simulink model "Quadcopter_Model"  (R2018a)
settings: Solver=VariableStepAuto  StartTime=0.0  StopTime=runtime  FixedStep=0.001  RelTol=1e-3
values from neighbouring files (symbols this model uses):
  delta_T = [ 0,  0,  9.404e-04 ]    [modelParameters.m]    (also in rich_params.m = [ 0,  0,  1.176e-04 ])
  g = 9.81    [modelParameters.m]    (also in rich_params.m)
  height_controlled_o = (((Rm*If        + (((omega0_o * 2 * Rm * Kv * Kq      * Kd + 1)^2) - 1)/(4* Rm*Kv^2*Kq      * Kd))/Vb)*(Pmax - Pmin) + Pmin)    [modelParameters.m]    (also in rich_params.m)
  If = 0.3836    [modelParameters.m]    (also in rich_params.m = 0.39)
  Jreq = 4.2012e-05    [modelParameters.m]    (also in rich_params.m = 1.376e-05)
  Jxx = 0.0110    (= 0.011)    [modelParameters.m]    (also in rich_params.m = 0.0081)
  Jyy = 0.0116    [modelParameters.m]    (also in rich_params.m = 0.0074)
  Jzz = 0.0223    [modelParameters.m]    (also in rich_params.m = 0.0135)
  Kd = 1.4852e-07    [modelParameters.m]    (also in rich_params.m = 5.194e-07)
  Kh = 3.4574e-04    (= 0.00034574)    [modelParameters.m]    (also in rich_params.m)
  Kq = 96.3422    [modelParameters.m]    (also in rich_params.m = 110)
  Kt = 1.2007e-05    [modelParameters.m]    (also in rich_params.m = 7.3956e-06)
  Kv = 96.3422    [modelParameters.m]    (also in rich_params.m = 110)
  m = 1.216    [modelParameters.m]    (also in rich_params.m = 0.656)
  omega0_o = sqrt((m*g)/(4*Kt))    [modelParameters.m]    (also in rich_params.m)
  omega1_o = sqrt((m*g)/(4*Kt))    [modelParameters.m]    (also in rich_params.m)
  omega2_o = sqrt((m*g)/(4*Kt))    [modelParameters.m]    (also in rich_params.m)
  omega3_o = sqrt((m*g)/(4*Kt))    [modelParameters.m]    (also in rich_params.m)
  pitch_o = 0    [modelParameters.m]    (also in rich_params.m)
  pitchrate_o = 0    [modelParameters.m]    (also in rich_params.m)
  Pmax = 1    [modelParameters.m]    (also in rich_params.m)
  Pmin = 0    [modelParameters.m]    (also in rich_params.m)
  r_oc = [ 0 ; 0 ; 0 ]    [modelParameters.m]    (also in rich_params.m)
  rhx = 0.16    [modelParameters.m]    (also in rich_params.m = 0.115)
  rhy = 0.16    [modelParameters.m]    (also in rich_params.m = 0.115)
  rhz = 0.03    [modelParameters.m]    (also in rich_params.m = 0.04)
  Rm = 0.235    [modelParameters.m]    (also in rich_params.m = 0.19)
  roll_o = 0    [modelParameters.m]    (also in rich_params.m)
  rollrate_o = 0    [modelParameters.m]    (also in rich_params.m)
  signal_mixer = [ 1, -1, -1, -1    [modelParameters.m]    (also in rich_params.m)
  Tc = 0.01    [modelParameters.m]    (also in rich_params.m)
  Tq = 0.005    [modelParameters.m]    (also in rich_params.m)
  Vb = 12.3    [modelParameters.m]    (also in rich_params.m = 11.4)
  x_controlled_o = 0    [modelParameters.m]    (also in rich_params.m)
  x_o = 0    [modelParameters.m]    (also in rich_params.m)
  x_vel_o = 0    [modelParameters.m]    (also in rich_params.m)
  y_controlled_o = 0    [modelParameters.m]    (also in rich_params.m)
  y_o = 0    [modelParameters.m]    (also in rich_params.m)
  y_vel_o = 0    [modelParameters.m]    (also in rich_params.m)
  yaw_controlled_o = 0    [modelParameters.m]    (also in rich_params.m)
  yaw_o = 0    [modelParameters.m]    (also in rich_params.m)
  yawrate_o = 0    [modelParameters.m]    (also in rich_params.m)
  z_o = 0    [modelParameters.m]    (also in rich_params.m)
  z_vel_o = 0    [modelParameters.m]    (also in rich_params.m)
undefined symbols (not defined in the file or in its folder): lqr_K
libraries: simulink x16, Derivative x13, dsparch4 x3, vrlib x1
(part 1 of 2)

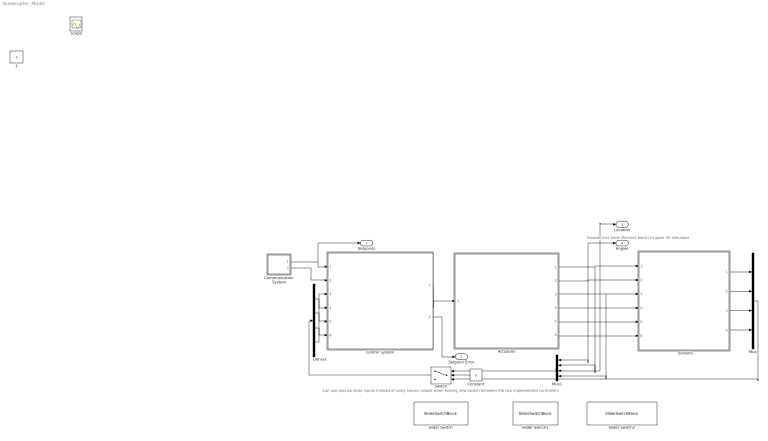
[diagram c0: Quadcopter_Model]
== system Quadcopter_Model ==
  note: Double-click here (Sensors block) to open 3D simulator
  note: Can use precise state inputs instead of noisy sensor values when testing new controls
  note: Switch between the two implemented controllers
  "     Sensors   " : Subsystem
  Actuation : Subsystem
  Communication System : Subsystem
  Constant : Constant  Value=0
  Control System : Subsystem
  Demux : Demux
  Mux : Mux
  Mux1 : Mux
  Slider Switch : SliderSwitchBlock  WebBlockId=752  LabelPosition=Hide
  Slider Switch1 : SliderSwitchBlock  WebBlockId=751  LabelPosition=Hide
  Slider Switch2 : SliderSwitchBlock  WebBlockId=769  LabelPosition=Hide
  Switch : Switch  Criteria=u2 ~= 0
  Setpoint Error : Outport  SignalName=setpoint_error
  Setpoints : Outport  Port=2
  Location : Outport  Port=3
  Angles : Outport  Port=4
  1 : Constant  IOType=siggen
  Scope : Scope
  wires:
  Control System/1(P) -> Actuation/1(P)
  Actuation/6(B_g) -> 1/6
  Actuation/5(B_vo_dot) -> 1/5
  Actuation/1(B_omega) -> Mux1/2, 1/1
  Actuation/2(euler_angles) -> Angles/1, 1/2, Mux1/1
  Communication System/1(Autonomous Setpoints) -> Control System/1(setpoints), Setpoints/1
  Actuation/3(B_vo) -> 1/3, Mux1/4
  1/2 -> Mux/2
  1/1 -> Mux/1
  1/3 -> Mux/3
  Mux/1 -> Switch/3
  Mux1/1 -> Switch/1
  Demux/4 -> Control System/3(velocity)
  Demux/3 -> Control System/6(current_position)
  Demux/2 -> Control System/5(euler_rates)
  Demux/1 -> Control System/4(euler_angles_filtered)
  Switch/1 -> Demux/1
  Constant/1 -> Switch/2
  1/4 -> Mux/4
  Actuation/4(E_ro) -> Location/1, 1/4, Mux1/3
  Control System/2(setpoint error) -> Setpoint Error/1
  Communication System/2(RC commands) -> Control System/2(RC Commands)

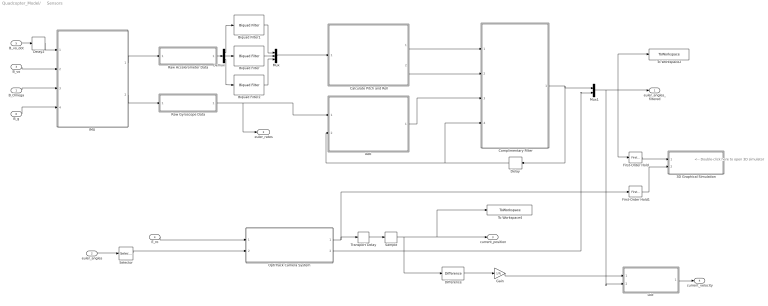
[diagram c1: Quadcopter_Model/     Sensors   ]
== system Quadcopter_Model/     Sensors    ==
  note: <-- Double-click here to open 3D simulator
  B_Omega : Inport
  euler_angles : Inport  Port=2
  B_vo : Inport  Port=3
  E_ro : Inport  Port=4
  B_vo_dot : Inport  Port=5
  B_g : Inport  Port=6
  3D Graphical Simulation : Subsystem
  "Aeb " : MATLAB Function  TreatAsAtomicUnit=on
  Biquad Filter : dsparch4/Biquad Filter  IIRFiltStruct=Direct form II  CoeffSource=Specify via dialog  BiQuadCoeffs=accel_SOS_Matrix  a0Flag=Warning  IC=0  ICnum=0  ICden=0  InputProcessing=Columns as channels (frame based)  denAccumFracLength=30  denProdOutputFracLength=30  secondMemoryFracLength=15  roundingMode=Floor  overflowMode=off  ScaleValues=1  optimizeScaleValues=on  ScaleValueMode=Specify via input port (g)  scaleValueFracLength=14  FilterSource=Specify via dialog  FilterObject=BQF
  Biquad Filter1 : dsparch4/Biquad Filter  IIRFiltStruct=Direct form II  CoeffSource=Specify via dialog  BiQuadCoeffs=accel_SOS_Matrix  a0Flag=Warning  IC=0  ICnum=0  ICden=0  InputProcessing=Columns as channels (frame based)  denAccumFracLength=30  denProdOutputFracLength=30  secondMemoryFracLength=15  roundingMode=Floor  overflowMode=off  ScaleValues=1  optimizeScaleValues=on  ScaleValueMode=Specify via input port (g)  scaleValueFracLength=14  FilterSource=Specify via dialog  FilterObject=BQF
  Biquad Filter2 : dsparch4/Biquad Filter  IIRFiltStruct=Direct form II  CoeffSource=Specify via dialog  BiQuadCoeffs=accel_SOS_Matrix  a0Flag=Warning  IC=0  ICnum=0  ICden=0  InputProcessing=Columns as channels (frame based)  denAccumFracLength=30  denProdOutputFracLength=30  secondMemoryFracLength=15  roundingMode=Floor  overflowMode=off  ScaleValues=1  optimizeScaleValues=on  ScaleValueMode=Specify via input port (g)  scaleValueFracLength=14  FilterSource=Specify via dialog  FilterObject=BQF
  Calculate Pitch and Roll : MATLAB Function  TreatAsAtomicUnit=on
  Complimentary Filter : MATLAB Function  TreatAsAtomicUnit=on
  Delay : Delay  DelayLength=1  InitialCondition=0
  Delay2 : Delay  DelayLength=1  InitialCondition=0  SampleTime=Tq
  Demux : Demux  Outputs=3
  Difference : simulink/Discrete/Difference  ICPrevInput=0.0  OutMin=[]  OutMax=[]  OutDataType=fixdt(1, 16)  OutScaling=2^-10  DoSatur=off
  First-Order Hold : simulink/Discrete/First-Order Hold  DisableCoverage=on  Ts=5e-3
  First-Order Hold1 : simulink/Discrete/First-Order Hold  DisableCoverage=on  Ts=5e-3
  Gain : Gain  Gain=1/Tc
  "IMU " : Subsystem
  "Lbe " : MATLAB Function  TreatAsAtomicUnit=on
  Mux : Mux  Inputs=3
  Mux1 : Mux  Inputs=2
  "OptiTrack Camera System " : Subsystem
  Raw Accelerometer Data : Subsystem  Variant=on
  Raw Gyroscope Data : Subsystem  Variant=on
  Sample : ZeroOrderHold  SampleTime=Tc
  Selector : Selector  InputPortWidth=3  IndexOptions=Index vector (dialog)  Indices=[3]  OutputSizes=1
  To Workspace2 : ToWorkspace  VariableName=angle_IMU_reading  SaveFormat=Structure With Time  SampleTime=Tq
  To Workspace4 : ToWorkspace  VariableName=position_model  SaveFormat=Structure With Time  SampleTime=Tc
  Transport Delay : TransportDelay  DelayTime=6e-3
  euler_angles_filtered : Outport
  euler_rates : Outport  Port=2
  current_position : Outport  Port=3
  current_velocity : Outport  Port=4
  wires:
  "IMU "/1(accelerometer) -> Raw Accelerometer Data/1(raw_accel_model)
  "IMU "/2(gyroscope) -> Raw Gyroscope Data/1(raw_gyro_model)
  B_vo/1 -> "IMU "/2(B_vo)
  B_Omega/1 -> "IMU "/3(B_Omega)
  B_g/1 -> "IMU "/4(B_g)
  Calculate Pitch and Roll/2(accel_roll) -> Complimentary Filter/2(accel_roll)
  Calculate Pitch and Roll/1(accel_pitch) -> Complimentary Filter/1(accel_pitch)
  First-Order Hold/1 -> 3D Graphical Simulation/1("Euler Angles ")
  E_ro/1 -> "OptiTrack Camera System "/1(E_ro)
  First-Order Hold1/1 -> 3D Graphical Simulation/2(Displacement)
  B_vo_dot/1 -> Delay2/1
  Delay2/1 -> "IMU "/1(B_vo_dot)
  "OptiTrack Camera System "/1(E_ro_camera) -> Transport Delay/1, First-Order Hold1/1
  Transport Delay/1 -> Sample/1
  Raw Gyroscope Data/1(raw_gyro) -> "Aeb "/1(gyro_reading), euler_rates/1
  Delay/1 -> Complimentary Filter/4(prev_euler_angles), "Aeb "/2(euler_angles_filtered)
  "OptiTrack Camera System "/2(yaw_camera) -> Mux1/2
  "Aeb "/1(euler_rates_IMU) -> Complimentary Filter/3(euler_rates_gyro)
  Raw Accelerometer Data/1(raw_accel) -> Demux/1
  Demux/2 -> Biquad Filter/1
  Demux/1 -> Biquad Filter1/1
  Demux/3 -> Biquad Filter2/1
  Biquad Filter/1 -> Mux/2
  Biquad Filter1/1 -> Mux/1
  Biquad Filter2/1 -> Mux/3
  Mux/1 -> Calculate Pitch and Roll/1(accel_reading)
  Complimentary Filter/1(euler_angles_IMU) -> Mux1/1, Delay/1
  euler_angles/1 -> Selector/1
  Selector/1 -> "OptiTrack Camera System "/2(yaw)
  Mux1/1 -> To Workspace2/1, First-Order Hold/1, euler_angles_filtered/1, "Lbe "/2(euler_angles)
  Difference/1 -> Gain/1
  Gain/1 -> "Lbe "/1(E_vo)
  "Lbe "/1(B_vo) -> current_velocity/1
  Sample/1 -> Difference/1, To Workspace4/1, current_position/1

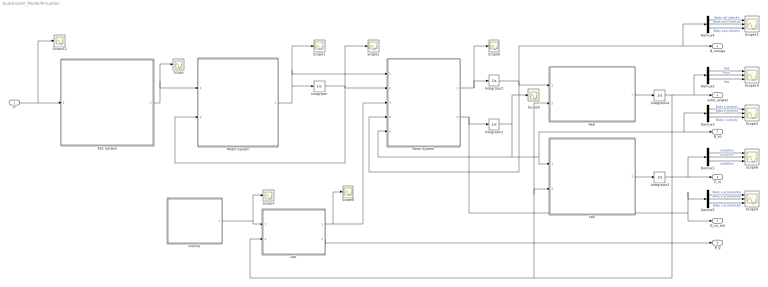
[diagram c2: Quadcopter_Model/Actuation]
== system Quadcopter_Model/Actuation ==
  P : Inport
  "Aeb " : MATLAB Function  TreatAsAtomicUnit=on
  Demux{1..5} (5 alike) : Demux  Outputs=3
  ESC System : MATLAB Function  TreatAsAtomicUnit=on
  "Gravity " : MATLAB Function  TreatAsAtomicUnit=on
  Integrator : Integrator  InitialCondition=[omega0_o, omega1_o, omega2_o, omega3_o]
  Integrator1 : Integrator  InitialCondition=[x_vel_o; y_vel_o; z_vel_o]
  Integrator2 : Integrator  InitialCondition=[rollrate_o; pitchrate_o; yawrate_o]
  Integrator3 : Integrator  InitialCondition=[x_o; y_o; z_o]
  Integrator4 : Integrator  InitialCondition=[roll_o; pitch_o; yaw_o]  ContinuousStateAttributes=['phi' 'theta' 'psi']
  "Lbe " : MATLAB Function  TreatAsAtomicUnit=on
  "Lbe " : MATLAB Function  TreatAsAtomicUnit=on
  Motor System : MATLAB Function  TreatAsAtomicUnit=on
  "Rotor System " : MATLAB Function  TreatAsAtomicUnit=on
  Scope{,1..2,5,7..9,12} (8 alike) : Scope
  Scope{3..4,6,10..11} (5 alike) : Scope  NumInputPorts=3
  B_omega : Outport
  euler_angles : Outport  Port=2
  B_vo : Outport  Port=3
  E_ro : Outport  Port=4
  B_vo_dot : Outport  Port=5
  B_g : Outport  Port=6
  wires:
  ESC System/1(Vb_eff) -> Scope/1, Motor System/1(Vb_eff)
  "Rotor System "/1(B_omega_dot) -> Scope9/1, Integrator2/1
  Integrator2/1 -> "Rotor System "/4(B_omega), B_omega/1, Demux4/1, "Aeb "/1(B_omega)
  "Aeb "/1(euler_rates) -> Integrator4/1
  "Lbe "/1(E_ro) -> Integrator3/1
  Integrator3/1 -> Demux1/1, E_ro/1
  "Lbe "/1(B_Fg) -> Scope8/1, "Rotor System "/3(B_Fg)
  "Lbe "/2(B_g) -> B_g/1
  Demux1/2 -> Scope6/2  "y position"
  Demux1/1 -> Scope6/1  "x position"
  Demux1/3 -> Scope6/3  "z position"
  Demux2/2 -> Scope10/2  "Pitch"
  Demux2/1 -> Scope10/1  "Roll"
  Demux2/3 -> Scope10/3  "Yaw"
  Demux4/2 -> Scope11/2  "Body pitch velocity"
  Demux4/1 -> Scope11/1  "Body roll velocity"
  Demux4/3 -> Scope11/3  "Body yaw velocity"
  Demux3/2 -> Scope3/2  "Body y velocity"
  Demux3/1 -> Scope3/1  "Body x velocity"
  Demux3/3 -> Scope3/3  "Body z velocity"
  Demux5/2 -> Scope4/2  "Body y acceleration"
  Demux5/1 -> Scope4/1  "Body x acceleration"
  Demux5/3 -> Scope4/3  "Body z acceleration"
  Integrator1/1 -> Scope5/1, "Rotor System "/5(B_vo), "Lbe "/1(B_vo), Demux3/1, B_vo/1
  "Rotor System "/2(B_vo_dot) -> Demux5/1, B_vo_dot/1, Integrator1/1
  Integrator4/1 -> euler_angles/1, Demux2/1, "Lbe "/2(euler_angles), "Aeb "/2(euler_angles), "Lbe "/2(euler_angles)
  P/1 -> Scope12/1, ESC System/1(P)
  "Gravity "/1(E_Fg) -> Scope7/1, "Lbe "/1(E_Fg)
  Integrator/1 -> Motor System/2(w), "Rotor System "/2(w), Scope2/1
  Motor System/1(w_dot) -> Integrator/1, Scope1/1, "Rotor System "/1(w_dot)

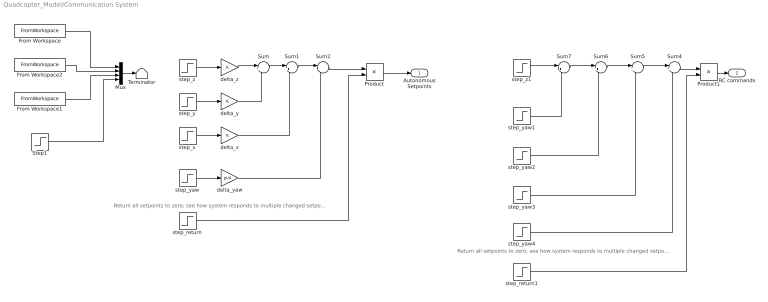
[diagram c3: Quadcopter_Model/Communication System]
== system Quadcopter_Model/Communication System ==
  note: Return all setpoints to zero; see how system responds to multiple changed setpoints
  note: Return all setpoints to zero; see how system responds to multiple changed setpoints
  From Workspace : FromWorkspace  Commented=on  VariableName=x_setpoint_model  SampleTime=Tq  Interpolate=off  OutputAfterFinalValue=Holding final value
  From Workspace1 : FromWorkspace  Commented=on  VariableName=z_setpoint_model  SampleTime=Tq  Interpolate=off  OutputAfterFinalValue=Holding final value
  From Workspace2 : FromWorkspace  Commented=on  VariableName=y_setpoint_model  SampleTime=Tq  Interpolate=off  OutputAfterFinalValue=Holding final value
  Mux : Mux  Commented=on
  Product : Product
  Product1 : Product
  Step1 : Step  Commented=on  After=0  SampleTime=0
  Sum{,1..2,4..7} (7 alike) : Sum  Inputs=|++
  Terminator : Terminator
  delta_x : Gain
  delta_y : Gain
  delta_yaw : Gain  Gain=pi/4
  delta_z : Gain
  step_return : Step  Time=30  Before=[1,1,1,1]  After=[0,0,0,0]  SampleTime=0
  step_return1 : Step  Time=35  Before=[1,1,1,1]  After=[0,0,0,0]  SampleTime=0
  step_x : Step  Time=18  Before=[0,0,0,0]  After=[1,0,0,0]  SampleTime=0
  step_y : Step  Time=12  Before=[0,0,0,0]  After=[0,1,0,0]  SampleTime=0
  step_yaw : Step  Time=25  Before=[0,0,0,0]  After=[0,0,0,1]  SampleTime=0
  step_yaw1 : Step  Time=15  Before=[0,0,0,0]  After=[0,0,0,1]  SampleTime=0
  step_yaw2 : Step  Time=20  Before=[0,0,0,0]  After=[0,0,0,-1]  SampleTime=0
  step_yaw3 : Step  Time=25  Before=[0,0,0,0]  After=[0,0,0,-1]  SampleTime=0
  step_yaw4 : Step  Time=30  Before=[0,0,0,0]  After=[0,0,0,1]  SampleTime=0
  step_z : Step  Time=5  Before=[0,0,0,0]  After=[0,0,-1,0]  SampleTime=0
  step_z1 : Step  Time=10  Before=[0,0,0,0]  After=[0,0,-2,0]  SampleTime=0
  Autonomous Setpoints : Outport
  RC commands : Outport  Port=2
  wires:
  From Workspace/1 -> Mux/1
  From Workspace2/1 -> Mux/2
  From Workspace1/1 -> Mux/3
  Step1/1 -> Mux/4
  step_z/1 -> delta_z/1
  step_y/1 -> delta_y/1
  Sum/1 -> Sum1/1
  step_x/1 -> delta_x/1
  step_yaw/1 -> delta_yaw/1
  Sum1/1 -> Sum2/1
  delta_yaw/1 -> Sum2/2
  Mux/1 -> Terminator/1
  Product/1 -> Autonomous Setpoints/1
  Sum2/1 -> Product/1
  step_return/1 -> Product/2
  Product1/1 -> RC commands/1
  step_return1/1 -> Product1/2
  Sum4/1 -> Product1/1
  Sum5/1 -> Sum4/1
  Sum6/1 -> Sum5/1
  Sum7/1 -> Sum6/1
  step_yaw1/1 -> Sum7/2
  step_yaw2/1 -> Sum6/2
  step_yaw4/1 -> Sum4/2
  step_yaw3/1 -> Sum5/2
  step_z1/1 -> Sum7/1
  delta_x/1 -> Sum1/2
  delta_y/1 -> Sum/2
  delta_z/1 -> Sum/1

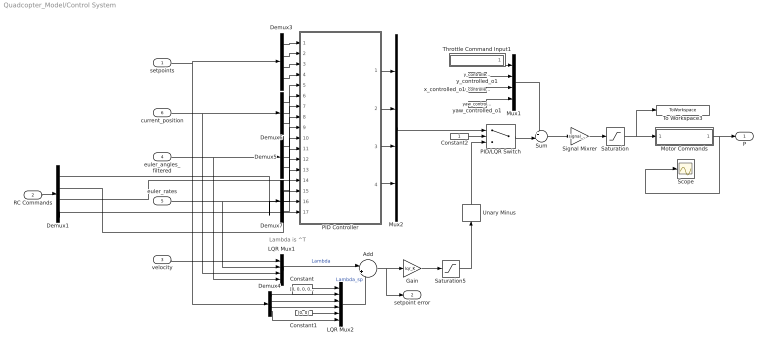
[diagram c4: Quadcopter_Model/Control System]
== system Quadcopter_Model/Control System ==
  note: Lambda is ^T
  setpoints : Inport
  RC Commands : Inport  Port=2
  velocity : Inport  Port=3
  euler_angles_filtered : Inport  Port=4
  euler_rates : Inport  Port=5
  current_position : Inport  Port=6
  Add : Sum  Inputs=|+-
  Constant : Constant  Value=[0, 0, 0, 0, 0, 0]
  Constant1 : Constant  Value=[0, 0]
  Constant2 : Constant
  Demux1 : Demux
  Demux3 : Demux
  Demux4 : Demux
  Demux5 : Demux  Outputs=3
  Demux6 : Demux  Outputs=3
  Demux7 : Demux  Outputs=3
  Gain : Gain  Gain=lqr_K  Multiplication=Matrix(K*u)
  LQR Mux1 : Mux
  LQR Mux2 : Mux  Inputs=6
  Motor Commands : Subsystem  Variant=on
  Mux1 : Mux
  Mux2 : Mux
  PID Controller : Subsystem
  PID/LQR Switch : Switch  Criteria=u2 ~= 0
  Saturation : Saturate  UpperLimit=Pmax*ones(4,1)  LowerLimit=Pmin*ones(4,1)
  Saturation5 : Saturate  UpperLimit=[20000, 20000, 20000, 20000]  LowerLimit=[-20000, -20000, -20000, -20000]
  Scope : Scope
  Signal Mixrer : Gain  Gain=signal_mixer  Multiplication=Matrix(K*u)
  Sum : Sum  Inputs=++|
  Throttle Command Input1 : Subsystem  Variant=on
  To Workspace3 : ToWorkspace  VariableName=motorCommands  SaveFormat=Structure With Time  SampleTime=Tq
  Unary Minus : UnaryMinus
  x_controlled_o1 : Constant  Value=x_controlled_o
  y_controlled_o1 : Constant  Value=y_controlled_o
  yaw_controlled_o1 : Constant  Value=yaw_controlled_o
  P : Outport
  setpoint error : Outport  Port=2
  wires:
  Motor Commands/1(z_command) -> P/1, Scope/1
  Saturation/1 -> To Workspace3/1, Motor Commands/1(z_command_model)
  setpoints/1 -> Demux3/1, Demux4/1
  current_position/1 -> Demux6/1, LQR Mux1/3
  euler_angles_filtered/1 -> LQR Mux1/4, Demux5/1
  euler_rates/1 -> Demux7/1, LQR Mux1/2
  Demux3/1 -> PID Controller/1(x_setpoint)
  Demux3/2 -> PID Controller/2(y_setpoint)
  Demux3/3 -> PID Controller/3(z_setpoint)
  Demux3/4 -> PID Controller/4(yaw_setpoint)
  Demux6/1 -> PID Controller/5(x_position)
  Demux6/2 -> PID Controller/6(y_position)
  Demux5/2 -> PID Controller/9(pitch)
  Demux5/3 -> PID Controller/10(yaw)
  Demux7/1 -> PID Controller/11(roll_rate)
  Demux7/2 -> PID Controller/12(pitch_rate)
  PID Controller/1(height_controlled) -> Mux2/1
  PID Controller/2(y_controlled) -> Mux2/2
  PID Controller/3(x_controlled) -> Mux2/3
  PID Controller/4(yaw_controlled) -> Mux2/4
  Mux2/1 -> PID/LQR Switch/1
  Demux4/1 -> LQR Mux2/2
  Demux4/2 -> LQR Mux2/3
  Demux4/3 -> LQR Mux2/4
  Demux4/4 -> LQR Mux2/6
  Constant/1 -> LQR Mux2/1
  Constant1/1 -> LQR Mux2/5
  LQR Mux1/1 -> Add/1  "Lambda"
  LQR Mux2/1 -> Add/2  "Lambda_sp"
  Demux7/3 -> PID Controller/13(yaw_rate)
  Demux5/1 -> PID Controller/8(roll)
  Demux6/3 -> PID Controller/7(z_position)
  Gain/1 -> Saturation5/1
  Saturation5/1 -> Unary Minus/1
  Unary Minus/1 -> PID/LQR Switch/3
  yaw_controlled_o1/1 -> Mux1/4
  x_controlled_o1/1 -> Mux1/3
  y_controlled_o1/1 -> Mux1/2
  Throttle Command Input1/1(z_command) -> Mux1/1
  PID/LQR Switch/1 -> Sum/2
  Signal Mixrer/1 -> Saturation/1
  Sum/1 -> Signal Mixrer/1
  Mux1/1 -> Sum/1
  Constant2/1 -> PID/LQR Switch/2
  Add/1 -> setpoint error/1, Gain/1
  velocity/1 -> LQR Mux1/1
  Demux1/4 -> PID Controller/17(RC_Yaw)
  Demux1/3 -> PID Controller/14(RC_Z)
  Demux1/2 -> PID Controller/15(RC_Roll)
  Demux1/1 -> PID Controller/16(RC_Pitch)
  RC Commands/1 -> Demux1/1

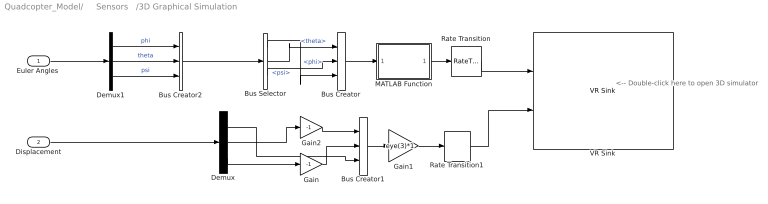
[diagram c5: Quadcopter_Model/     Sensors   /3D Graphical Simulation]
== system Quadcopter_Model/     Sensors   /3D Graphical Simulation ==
  note: <-- Double-click here to open 3D simulator
  "Euler Angles " : Inport
  Displacement : Inport  Port=2
  Bus Creator : BusCreator  Inputs=3
  Bus Creator1 : BusCreator  Inputs=3
  Bus Creator2 : BusCreator  Inputs=3
  Bus Selector : BusSelector  OutputSignals=phi,theta,psi
  Demux : Demux  Outputs=3
  Demux1 : Demux  Outputs=3
  Gain : Gain  Gain=-1
  Gain1 : Gain  Gain=eye(3)*1  Multiplication=Matrix(K*u)
  Gain2 : Gain  Gain=-1
  MATLAB Function : MATLAB Function  TreatAsAtomicUnit=on
  Rate Transition : RateTransition  OutPortSampleTime=0.06
  Rate Transition1 : RateTransition  OutPortSampleTime=0.06
  VR Sink : vrlib/VR Sink  InstantiateOnLoad=on  SampleTime=-1  ViewEnable=on  RemoteChange=off  RemoteView=off  FieldsWritten=Helicopter.rotation.4.1.1.double#Helicopter.translation.3.1.1.double  WorldFileName=quadrotor_world_ucart.wrl  AutoView=on  VideoDimensions=[]  AllowVariableSize=off  FigureProperties={'Position', 'Name', 'Viewpoint', 'CameraBound', 'CameraDirection', 'CameraPosition', 'CameraUpVector', 'ZoomFactor', 'Antialiasing', 'Headlight', 'Lighting', 'NavPanel', 'Sound', 'StatusBar', 'Stereo3D', 'Stereo3DCameraOffset', 'Stereo3DHIT', 'ToolBar', 'Textures', 'Transparency', 'Triad', 'Wireframe', 'NavZones', 'NavMode', 'NavSpeed', 'CaptureFileFormat', 'CaptureFileName', 'Record2DCompressMet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
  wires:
  Bus Creator2/1 -> Bus Selector/1
  Demux/1 -> Bus Creator1/3
  Gain/1 -> Bus Creator1/2
  Gain2/1 -> Bus Creator1/1
  Rate Transition1/1 -> VR Sink/2
  Rate Transition/1 -> VR Sink/1
  Demux/3 -> Gain/1
  Demux/2 -> Gain2/1
  Bus Creator1/1 -> Gain1/1
  Bus Selector/1 -> Bus Creator/3  "<phi>"
  Bus Selector/3 -> Bus Creator/2  "<psi>"
  Bus Selector/2 -> Bus Creator/1  "<theta>"
  Gain1/1 -> Rate Transition1/1
  Demux1/3 -> Bus Creator2/3  "psi"
  Demux1/2 -> Bus Creator2/2  "theta"
  Demux1/1 -> Bus Creator2/1  "phi"
  Bus Creator/1 -> MATLAB Function/1(u)
  MATLAB Function/1(y) -> Rate Transition/1
  Displacement/1 -> Demux/1
  "Euler Angles "/1 -> Demux1/1

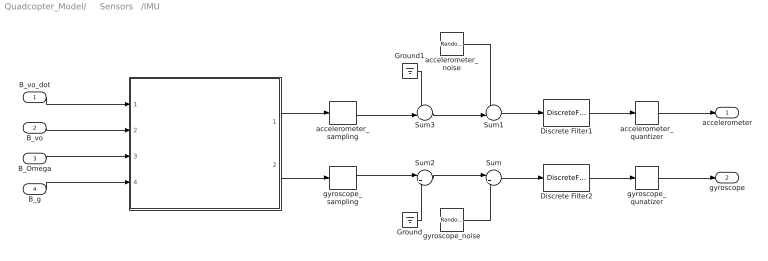
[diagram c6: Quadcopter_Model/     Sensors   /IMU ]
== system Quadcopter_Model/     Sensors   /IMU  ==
  B_vo_dot : Inport
  B_vo : Inport  Port=2
  B_Omega : Inport  Port=3
  B_g : Inport  Port=4
  " " : MATLAB Function  TreatAsAtomicUnit=on
  Discrete Filter1 : DiscreteFilter  Numerator=[0 0.749]  Denominator=[1 -0.251]  InitialStates=[0, 0, -1]  SampleTime=Tq
  Discrete Filter2 : DiscreteFilter  Numerator=[0 0.7327]  Denominator=[1 -0.2673]  SampleTime=Tq
  Ground : Ground
  Ground1 : Ground
  Sum : Sum  Inputs=|++
  Sum1 : Sum  Inputs=++|
  Sum2 : Sum  Inputs=|++
  Sum3 : Sum  Inputs=++|
  accelerometer_noise : RandomNumber  Mean=zeros(3,1)  Variance=[ 3e-7 ; 3.3e-7 ; 7.2e-7 ]  Seed=[0,1,2]  SampleTime=Tq
  accelerometer_quantizer : Quantizer  QuantizationInterval=2.4400e-04
  accelerometer_sampling : ZeroOrderHold  SampleTime=Tq
  gyroscope_noise : RandomNumber  Mean=zeros(3,1)  Variance=[ 2.2e-8 ; 1.1e-7 ; 2.4e-8 ]  Seed=[0,1,2]  SampleTime=Tq
  gyroscope_qunatizer : Quantizer  QuantizationInterval=1.1e-3
  gyroscope_sampling : ZeroOrderHold  SampleTime=Tq
  accelerometer : Outport
  gyroscope : Outport  Port=2
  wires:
  accelerometer_noise/1 -> Sum1/1
  Sum2/1 -> Sum/1
  Sum3/1 -> Sum1/2
  gyroscope_noise/1 -> Sum/2
  gyroscope_sampling/1 -> Sum2/1
  accelerometer_sampling/1 -> Sum3/2
  Ground/1 -> Sum2/2
  Ground1/1 -> Sum3/1
  B_vo_dot/1 -> " "/1(B_vo_dot)
  B_vo/1 -> " "/2(B_vo)
  B_Omega/1 -> " "/3(B_Omega)
  B_g/1 -> " "/4(B_g)
  " "/2(gyroReading) -> gyroscope_sampling/1
  " "/1(accelReading) -> accelerometer_sampling/1
  Sum1/1 -> Discrete Filter1/1
  Sum/1 -> Discrete Filter2/1
  accelerometer_quantizer/1 -> accelerometer/1
  gyroscope_qunatizer/1 -> gyroscope/1
  Discrete Filter1/1 -> accelerometer_quantizer/1
  Discrete Filter2/1 -> gyroscope_qunatizer/1

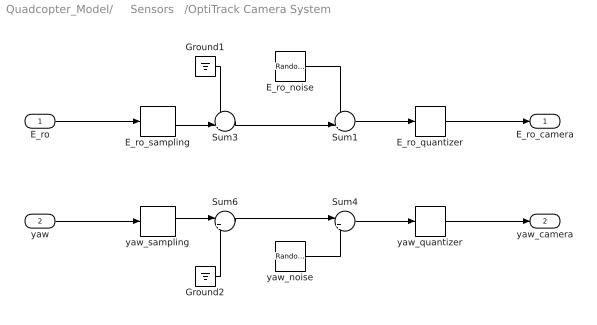
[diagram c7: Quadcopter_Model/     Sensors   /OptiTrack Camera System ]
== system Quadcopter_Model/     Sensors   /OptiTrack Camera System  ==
  E_ro : Inport
  yaw : Inport  Port=2
  E_ro_noise : RandomNumber  Mean=zeros(3,1)  Variance=[ 7.9664e-10 ; 1.1928e-10 ; 5.0636e-10 ]  Seed=[0,1,2]  SampleTime=Tc
  E_ro_quantizer : Quantizer  QuantizationInterval=2.4400e-04
  E_ro_sampling : ZeroOrderHold  SampleTime=Tc
  Ground1 : Ground
  Ground2 : Ground
  Sum1 : Sum  Inputs=++|
  Sum3 : Sum  Inputs=++|
  Sum4 : Sum  Inputs=|++
  Sum6 : Sum  Inputs=|++
  yaw_noise : RandomNumber  Variance=1.0783e-9  SampleTime=Tq
  yaw_quantizer : Quantizer  QuantizationInterval=1.1e-3
  yaw_sampling : ZeroOrderHold  SampleTime=Tq
  E_ro_camera : Outport
  yaw_camera : Outport  Port=2
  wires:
  E_ro_noise/1 -> Sum1/1
  Sum3/1 -> Sum1/2
  Sum1/1 -> E_ro_quantizer/1
  E_ro_sampling/1 -> Sum3/2
  Ground1/1 -> Sum3/1
  Sum4/1 -> yaw_quantizer/1
  Sum6/1 -> Sum4/1
  yaw_noise/1 -> Sum4/2
  yaw_sampling/1 -> Sum6/1
  Ground2/1 -> Sum6/2
  yaw/1 -> yaw_sampling/1
  E_ro/1 -> E_ro_sampling/1
  E_ro_quantizer/1 -> E_ro_camera/1
  yaw_quantizer/1 -> yaw_camera/1

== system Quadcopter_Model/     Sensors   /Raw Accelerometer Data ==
  note: 1) Add Subsystem or Model blocks as valid variant choices. 2) You cannot connect blocks at this level. At simulation, connectivity is automatically determined, based on the active variant and port name matching.
  raw_accel_model : Inport
  Feedback : Subsystem  VariantControl=logAnalysisToggle==0
  "Raw Accelerometer Data " : Subsystem  VariantControl=logAnalysisToggle==1
  raw_accel : Outport

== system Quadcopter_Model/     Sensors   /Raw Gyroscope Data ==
  note: 1) Add Subsystem or Model blocks as valid variant choices. 2) You cannot connect blocks at this level. At simulation, connectivity is automatically determined, based on the active variant and port name matching.
  raw_gyro_model : Inport
  Feedback : Subsystem  VariantControl=logAnalysisToggle==0
  "Raw Gyroscope Data " : Subsystem  VariantControl=logAnalysisToggle==1
  raw_gyro : Outport

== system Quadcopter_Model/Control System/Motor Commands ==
  note: 1) Add Subsystem or Model blocks as valid variant choices. 2) You cannot connect blocks at this level. At simulation, connectivity is automatically determined, based on the active variant and port name matching.
  z_command_model : Inport
  Feedback : Subsystem  VariantControl=logAnalysisToggle==0
  Motor Command : Subsystem  VariantControl=logAnalysisToggle==1
  z_command : Outport

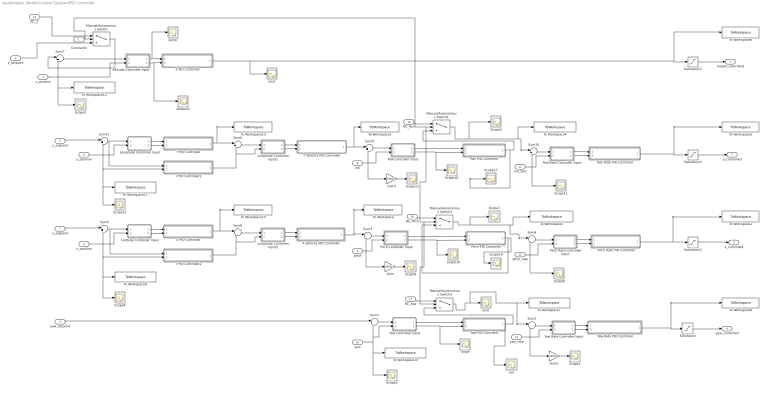
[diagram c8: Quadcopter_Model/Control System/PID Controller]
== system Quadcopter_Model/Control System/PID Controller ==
  x_setpoint : Inport
  y_setpoint : Inport  Port=2
  z_setpoint : Inport  Port=3
  yaw_setpoint : Inport  Port=4
  x_position : Inport  Port=5
  y_position : Inport  Port=6
  z_position : Inport  Port=7
  roll : Inport  Port=8
  pitch : Inport  Port=9
  yaw : Inport  Port=10
  roll_rate : Inport  Port=11
  pitch_rate : Inport  Port=12
  yaw_rate : Inport  Port=13
  RC_Z : Inport  Port=14
  RC_Roll : Inport  Port=15
  RC_Pitch : Inport  Port=16
  RC_Yaw : Inport  Port=17
  Altitude Controller Input : Subsystem  Variant=on
  Constant1 : Constant
  Gain : Gain  Gain=180/pi
  Gain1 : Gain  Gain=180/pi
  Gain2 : Gain  Gain=180/pi
  Latitude Controller Input : Subsystem  Variant=on
  Longitude Controller Input : Subsystem  Variant=on
  Longitude Controller Input1 : Subsystem  Variant=on
  Longitude Controller Input2 : Subsystem  Variant=on
  Manual/Autonomous Switch{,1..3} (4 alike) : Switch  Criteria=u2 ~= 0
  Pitch Controller Input : Subsystem  Variant=on
  Pitch PID Controller : Subsystem  mask{Kp=35, Ki=0, Kd=1, a=0.88, Ts=Tq}
      mask prompts: a "alpha"; Ts "Sample Time"
  Pitch Rate Controller Input : Subsystem  Variant=on
  Pitch Rate PID Controller : Subsystem  mask{Kp=0.03, Ki=0, Kd=0.005, a=0.88, Ts=Tq}
      mask prompts: a "alpha"; Ts "Sample Time"
  Roll Controller Input : Subsystem  Variant=on
  Roll PID Controller : Subsystem  mask{Kp=35, Ki=0, Kd=1, a=0.88, Ts=Tq}
      mask prompts: a "alpha"; Ts "Sample Time"
  Roll Rate Controller Input : Subsystem  Variant=on
  Roll Rate PID Controller : Subsystem  mask{Kp=0.03, Ki=0, Kd=0.005, a=0.88, Ts=Tq}
      mask prompts: a "alpha"; Ts "Sample Time"
  Saturation{,1..3} (4 alike) : Saturate  UpperLimit=20000  LowerLimit=-20000
  Scope{1..7,9,11..13,16..19} (15 alike) : Scope
  Sum{1..11} (11 alike) : Sum  Inputs=|+-
  To Workspace : ToWorkspace  VariableName=pitch_setpoint_model  SaveFormat=Structure With Time  SampleTime=-1
  To Workspace1 : ToWorkspace  VariableName=pitchrate_setpoint_model  SaveFormat=Structure With Time  SampleTime=Tq
  To Workspace10 : ToWorkspace  VariableName=yaw_value_model  SaveFormat=Structure With Time  SampleTime=Tc
  To Workspace11 : ToWorkspace  VariableName=y_position_model  SaveFormat=Structure With Time  SampleTime=Tc
  To Workspace12 : ToWorkspace  VariableName=z_position_model  SaveFormat=Structure With Time  SampleTime=Tc
  To Workspace13 : ToWorkspace  VariableName=y_vel_setpoint_model  SaveFormat=Structure With Time  SampleTime=Tc
  To Workspace14 : ToWorkspace  VariableName=x_vel_setpoint_model  SaveFormat=Structure With Time  SampleTime=Tc
  To Workspace2 : ToWorkspace  VariableName=x_command_model  SaveFormat=Structure With Time  SampleTime=Tq
  To Workspace3 : ToWorkspace  VariableName=roll_setpoint_model  SaveFormat=Structure With Time  SampleTime=Tc
  To Workspace4 : ToWorkspace  VariableName=rollrate_setpoint_model  SaveFormat=Structure With Time  SampleTime=Tq
  To Workspace5 : ToWorkspace  VariableName=y_command_model  SaveFormat=Structure With Time  SampleTime=Tq
  To Workspace6 : ToWorkspace  VariableName=z_command_model  SaveFormat=Structure With Time  SampleTime=Tc
  To Workspace7 : ToWorkspace  VariableName=yawrate_setpoint_model  SaveFormat=Structure With Time  SampleTime=Tc
  To Workspace8 : ToWorkspace  VariableName=yaw_command_model  SaveFormat=Structure With Time  SampleTime=Tq
  To Workspace9 : ToWorkspace  VariableName=x_position_model  SaveFormat=Structure With Time  SampleTime=Tc
  X PID Controller : Subsystem  mask{Kp=0.55, Ki=0.0075, Kd=0, a=0.88, Ts=Tc}
      mask prompts: a "alpha"; Ts "Sample Time"
  X Velocity PID Controller : Subsystem  mask{Kp=-0.1, Ki=0, Kd=-0.02, a=0.00, Ts=Tc}
      mask prompts: a "alpha"; Ts "Sample Time"
  Y PID Controller : Subsystem  mask{Kp=0.55, Ki=0.0075, Kd=0, a=0.88, Ts=Tc}
      mask prompts: a "alpha"; Ts "Sample Time"
  Y PID Controller1 : Subsystem  mask{Kp=0, Ki=0, Kd=-1, a=0.88, Ts=Tc}
      mask prompts: a "alpha"; Ts "Sample Time"
  Y PID Controller2 : Subsystem  mask{Kp=0, Ki=0, Kd=-1, a=0.88, Ts=Tc}
      mask prompts: a "alpha"; Ts "Sample Time"
  Y Velocity PID Controller : Subsystem  mask{Kp=0.1, Ki=0, Kd=0.02, a=0.00, Ts=Tc}
      mask prompts: a "alpha"; Ts "Sample Time"
  Yaw Controller Input : Subsystem  Variant=on
  Yaw PID Controller : Subsystem  mask{Kp=2.6, Ki=0, Kd=0, a=0.88, Ts=Tc}
      mask prompts: a "alpha"; Ts "Sample Time"
  Yaw Rate Controller Input : Subsystem  Variant=on
  Yaw Rate PID Controller : Subsystem  mask{Kp=0.297, Ki=0, Kd=0, a=0.88, Ts=Tq}
      mask prompts: a "alpha"; Ts "Sample Time"
  Z PID Controller : Subsystem  mask{Kp=-0.098040, Ki=-0.00817, Kd=-0.07353, a=0.88, Ts=Tc}
      mask prompts: a "alpha"; Ts "Sample Time"
  angle : Scope
  error : Scope
  out : Scope
  zerror : Scope
  "zout " : Scope
  zposition : Scope
  height_controlled : Outport
  y_controlled : Outport  Port=2
  x_controlled : Outport  Port=3
  yaw_controlled : Outport  Port=4
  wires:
  pitch_rate/1 -> Pitch Rate Controller Input/2(pitchrate_model), Scope6/1, Sum4/2
  z_setpoint/1 -> Manual/Autonomous Switch/3
  x_position/1 -> Sum5/2, Latitude Controller Input/2(x_position_model), Scope4/1, To Workspace9/1, Y PID Controller2/2(x_pos)
  Pitch PID Controller/1(pitchrate_setpoint) -> Manual/Autonomous Switch2/3, Scope19/1
  pitch/1 -> Pitch Controller Input/2(pitch_angle_model), Gain/1, Sum3/2
  Gain/1 -> Scope9/1
  Yaw Rate PID Controller/1(yaw_motor_command) -> To Workspace8/1, Saturation/1
  Pitch Rate PID Controller/1(x_motor_command) -> Saturation1/1, To Workspace2/1
  x_setpoint/1 -> Sum5/1
  roll_rate/1 -> Roll Rate Controller Input/2(rollrate_model), Scope11/1, Sum10/2
  Roll PID Controller/1(rollrate_setpoint) -> Scope17/1, Manual/Autonomous Switch1/3
  roll/1 -> Roll Controller Input/2(roll_angle_model), Gain2/1, Sum9/2
  Gain2/1 -> Scope13/1
  y_setpoint/1 -> Sum11/1
  yaw/1 -> Yaw Controller Input/2(yaw_angle_model), Sum1/2, Scope3/1, To Workspace10/1
  yaw_setpoint/1 -> Sum1/1
  yaw_rate/1 -> Gain1/1, Yaw Rate Controller Input/2(yawrate_model), Sum2/2
  Gain1/1 -> Scope1/1
  Yaw PID Controller/1(yawrate_setpoint) -> out/1, Manual/Autonomous Switch3/3
  z_position/1 -> Altitude Controller Input/2(z_position_model), To Workspace12/1, Scope2/1, Sum7/2
  Sum1/1 -> Yaw Controller Input/1(yaw_error_model)
  Sum2/1 -> Yaw Rate Controller Input/1(yawrate_error_model)
  Sum5/1 -> Latitude Controller Input/1(x_error_model), Y PID Controller2/1(x_error)
  Sum3/1 -> Pitch Controller Input/1(pitch_error_model)
  Sum4/1 -> Pitch Rate Controller Input/1(pitchrate_error_model)
  Sum9/1 -> Roll Controller Input/1(roll_error_model)
  Sum10/1 -> Roll Rate Controller Input/1(rollrate_error_model)
  Roll Rate PID Controller/1(y_motor_command) -> To Workspace5/1, Saturation2/1
  Saturation3/1 -> height_controlled/1
  Saturation2/1 -> y_controlled/1
  Saturation1/1 -> x_controlled/1
  Saturation/1 -> yaw_controlled/1
  Longitude Controller Input/2(y_position) -> Y PID Controller/2(y_pos)
  Longitude Controller Input/1(y_error) -> Y PID Controller/1(y_error)
  y_position/1 -> Longitude Controller Input/2(y_position_model), Y PID Controller1/2(y_pos), To Workspace11/1, Scope12/1, Sum11/2
  Latitude Controller Input/1(x_error) -> X PID Controller/1(x_error)
  Latitude Controller Input/2(x_position) -> X PID Controller/2(x_pos)
  Yaw Controller Input/2(yaw_angle) -> angle/1, Yaw PID Controller/2(yaw_angle)
  Altitude Controller Input/1(z_error) -> zerror/1, Z PID Controller/1(z_error)
  Altitude Controller Input/2(z_position) -> zposition/1, Z PID Controller/2(z_pos)
  Pitch Controller Input/2(pitch_angle) -> Scope18/1, Pitch PID Controller/2(pitch_angle)
  Yaw Rate Controller Input/1(yawrate_error) -> Yaw Rate PID Controller/1(yawrate_error)
  Yaw Rate Controller Input/2(yawrate) -> Yaw Rate PID Controller/2(yawrate)
  Pitch Rate Controller Input/1(pitchrate_error) -> Pitch Rate PID Controller/1(pitchrate_error)
  Pitch Rate Controller Input/2(pitchrate) -> Pitch Rate PID Controller/2(pitchrate)
  Roll Controller Input/2(roll_angle) -> Scope16/1, Roll PID Controller/2(roll_angle)
  Roll Rate Controller Input/1(rollrate_error) -> Roll Rate PID Controller/1(rollrate_error)
  Roll Rate Controller Input/2(rollrate) -> Roll Rate PID Controller/2(rollrate)
  Sum11/1 -> Longitude Controller Input/1(y_error_model), Y PID Controller1/1(y_error)
  Y PID Controller/1(roll_setpoint) -> To Workspace13/1, Sum6/1
  Y PID Controller1/1(y_vel_setpoint) -> Longitude Controller Input1/2(y_vel_model), Sum6/2
  Sum6/1 -> Longitude Controller Input1/1(y_vel_error_model)
  Longitude Controller Input1/1(y_vel_error) -> Y Velocity PID Controller/1(y_error)
  Longitude Controller Input1/2(y_vel) -> Y Velocity PID Controller/2(y_pos)
  X PID Controller/1(pitch_setpoint) -> To Workspace14/1, Sum8/1
  Y PID Controller2/1(x_vel_setpoint) -> Longitude Controller Input2/2(x_vel_model), Sum8/2
  Sum8/1 -> Longitude Controller Input2/1(x_vel_error_model)
  Longitude Controller Input2/1(x_vel_error) -> X Velocity PID Controller/1(x_vel_error)
  Longitude Controller Input2/2(x_vel) -> X Velocity PID Controller/2(x_vel)
  Z PID Controller/1(z_motor_command) -> "zout "/1, To Workspace6/1, Saturation3/1
  Y Velocity PID Controller/1(roll_setpoint) -> To Workspace3/1, Sum9/1
  X Velocity PID Controller/1(pitch_setpoint) -> To Workspace/1, Sum3/1
  Roll Controller Input/1(roll_error) -> Roll PID Controller/1(roll_error)
  Manual/Autonomous Switch1/1 -> To Workspace4/1, Sum10/1, Scope5/1
  Pitch Controller Input/1(pitch_error) -> Pitch PID Controller/1(pitch_error)
  Manual/Autonomous Switch2/1 -> Sum4/1, To Workspace1/1, Scope7/1
  Constant1/1 -> Manual/Autonomous Switch3/2, Manual/Autonomous Switch2/2, Manual/Autonomous Switch1/2, Manual/Autonomous Switch/2
  Manual/Autonomous Switch3/1 -> Sum2/1, To Workspace7/1, error/1
  RC_Z/1 -> Manual/Autonomous Switch/1
  RC_Roll/1 -> Manual/Autonomous Switch1/1
  RC_Pitch/1 -> Manual/Autonomous Switch2/1
  RC_Yaw/1 -> Manual/Autonomous Switch3/1
  Sum7/1 -> Altitude Controller Input/1(z_error_model)
  Manual/Autonomous Switch/1 -> Sum7/1
  Yaw Controller Input/1(yaw_error) -> Yaw PID Controller/1(yaw_error)

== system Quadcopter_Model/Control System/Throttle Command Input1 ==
  note: 1) Add Subsystem or Model blocks as valid variant choices. 2) You cannot connect blocks at this level. At simulation, connectivity is automatically determined, based on the active variant and port name matching.
  Auto Takeoff : Subsystem  VariantControl=logAnalysisToggle==1
  height_controlled_o : Subsystem  VariantControl=logAnalysisToggle==0
  z_command : Outport

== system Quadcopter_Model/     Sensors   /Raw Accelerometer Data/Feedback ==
  raw_accel_model : Inport
  raw_accel : Outport
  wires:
  raw_accel_model/1 -> raw_accel/1

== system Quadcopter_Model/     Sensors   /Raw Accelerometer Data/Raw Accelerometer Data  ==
  From Workspace5 : FromWorkspace  VariableName=raw_accel_data  SampleTime=Tq
  raw_accel : Outport
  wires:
  From Workspace5/1 -> raw_accel/1

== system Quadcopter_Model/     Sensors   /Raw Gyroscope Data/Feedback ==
  raw_gyro_model : Inport
  raw_gyro : Outport
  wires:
  raw_gyro_model/1 -> raw_gyro/1

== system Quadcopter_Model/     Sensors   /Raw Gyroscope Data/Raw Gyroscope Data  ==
  From Workspace5 : FromWorkspace  VariableName=raw_gyro_data  SampleTime=Tq
  raw_gyro : Outport
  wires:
  From Workspace5/1 -> raw_gyro/1

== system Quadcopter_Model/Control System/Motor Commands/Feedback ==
  z_command_model : Inport
  z_command : Outport
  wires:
  z_command_model/1 -> z_command/1

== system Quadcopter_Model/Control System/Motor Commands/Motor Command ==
  From Workspace5 : FromWorkspace  VariableName=motor_commands  SampleTime=Tq
  z_command : Outport
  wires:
  From Workspace5/1 -> z_command/1

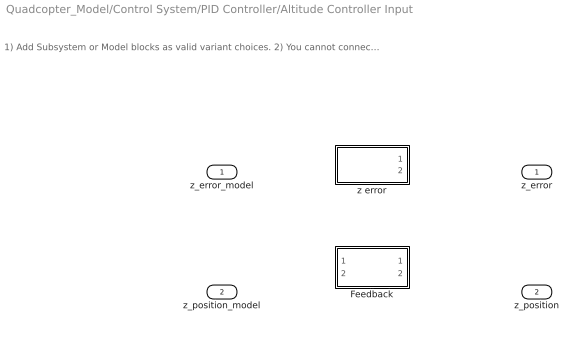
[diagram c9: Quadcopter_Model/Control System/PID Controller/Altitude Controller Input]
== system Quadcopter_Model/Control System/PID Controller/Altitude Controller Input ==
  note: 1) Add Subsystem or Model blocks as valid variant choices. 2) You cannot connect blocks at this level. At simulation, connectivity is automatically determined, based on the active variant and port name matching.
  z_error_model : Inport
  z_position_model : Inport  Port=2
  Feedback : Subsystem  VariantControl=logAnalysisToggle==0
  z error : Subsystem  VariantControl=logAnalysisToggle==1
  z_error : Outport
  z_position : Outport  Port=2

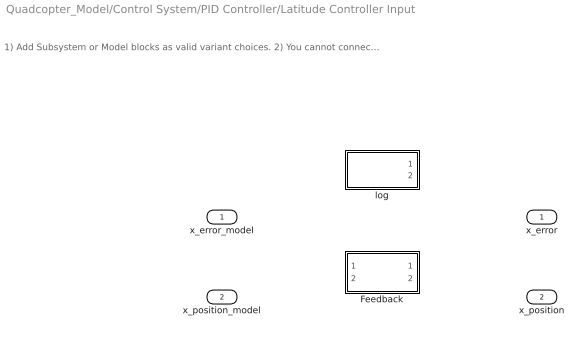
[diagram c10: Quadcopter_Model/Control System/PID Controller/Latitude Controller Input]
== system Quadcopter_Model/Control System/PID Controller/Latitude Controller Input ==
  note: 1) Add Subsystem or Model blocks as valid variant choices. 2) You cannot connect blocks at this level. At simulation, connectivity is automatically determined, based on the active variant and port name matching.
  x_error_model : Inport
  x_position_model : Inport  Port=2
  Feedback : Subsystem  VariantControl=logAnalysisToggle==0
  log : Subsystem  VariantControl=logAnalysisToggle==1
  x_error : Outport
  x_position : Outport  Port=2

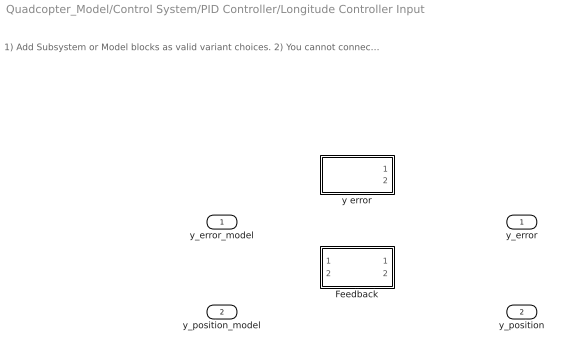
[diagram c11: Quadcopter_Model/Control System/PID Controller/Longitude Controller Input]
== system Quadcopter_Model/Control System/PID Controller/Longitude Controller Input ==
  note: 1) Add Subsystem or Model blocks as valid variant choices. 2) You cannot connect blocks at this level. At simulation, connectivity is automatically determined, based on the active variant and port name matching.
  y_error_model : Inport
  y_position_model : Inport  Port=2
  Feedback : Subsystem  VariantControl=logAnalysisToggle==0
  y error : Subsystem  VariantControl=logAnalysisToggle==1
  y_error : Outport
  y_position : Outport  Port=2

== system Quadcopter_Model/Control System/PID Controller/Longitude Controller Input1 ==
  note: 1) Add Subsystem or Model blocks as valid variant choices. 2) You cannot connect blocks at this level. At simulation, connectivity is automatically determined, based on the active variant and port name matching.
  y_vel_error_model : Inport
  y_vel_model : Inport  Port=2
  Feedback : Subsystem  VariantControl=logAnalysisToggle==0
  y error : Subsystem  VariantControl=logAnalysisToggle==1
  y_vel_error : Outport
  y_vel : Outport  Port=2

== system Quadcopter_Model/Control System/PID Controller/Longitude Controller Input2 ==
  note: 1) Add Subsystem or Model blocks as valid variant choices. 2) You cannot connect blocks at this level. At simulation, connectivity is automatically determined, based on the active variant and port name matching.
  x_vel_error_model : Inport
  x_vel_model : Inport  Port=2
  Feedback : Subsystem  VariantControl=logAnalysisToggle==0
  y error : Subsystem  VariantControl=logAnalysisToggle==1
  x_vel_error : Outport
  x_vel : Outport  Port=2

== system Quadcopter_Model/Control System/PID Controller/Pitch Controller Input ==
  note: 1) Add Subsystem or Model blocks as valid variant choices. 2) You cannot connect blocks at this level. At simulation, connectivity is automatically determined, based on the active variant and port name matching.
  pitch_error_model : Inport
  pitch_angle_model : Inport  Port=2
  Feedback : Subsystem  VariantControl=logAnalysisToggle==0
  pitch error : Subsystem  VariantControl=logAnalysisToggle==1
  pitch_error : Outport
  pitch_angle : Outport  Port=2

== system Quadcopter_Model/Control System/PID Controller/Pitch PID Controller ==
  pitch_error : Inport
  pitch_angle : Inport  Port=2
  Add : Sum  Inputs=+-
  Discrete D Controller : Derivative/Discrete D Controller  Kd=Kd  a=a
  Discrete PI Controller : simulink/Continuous/PID Controller  Controller=PI  TimeDomain=Discrete-time  SampleTime=Ts  IntegratorMethod=Forward Euler  FilterMethod=Forward Euler  Form=Parallel  UseFilter=on  ControllerParametersSource=internal  P=Kp  I=Ki  D=0  N=100  InitialConditionSource=internal  InitialConditionForIntegrator=0  InitialConditionForFilter=0  ExternalReset=none  LimitOutput=off  UpperSaturationLimit=inf  LowerSaturationLimit=-inf  LinearizeAsGain=off  AntiWindupMode=none  Kb=1  TrackingMode=off  Kt=1  PParamMin=[]  PParamMax=[]  IParamMin=[]  IParamMax=[]  DParamMin=[]  DParamMax=[]  NParamMin=[]  NParamMax=[]  KbParamMin=[]  KbParamMax=[]  KtParamMin=[]  KtParamMax=[]  POutMin=[]  POutMax=[]  IOutMin=[]  IOutMax=[]  DOutMin=[]  DOutMax=[]  NOutMin=[]  NOutMax=[]  KbOutMin=[]  KbOutMax=[]  KtOutMin=[]  KtOutMax=[]  IntegratorOutMin=[]  IntegratorOutMax=[]  FilterOutMin=[]  FilterOutMax=[]  SumOutMin=[]  SumOutMax=[]  SumI1OutMin=[]  SumI1OutMax=[]  SumI2OutMin=[]  SumI2OutMax=[]  SumI3OutMin=[]  SumI3OutMax=[]  SumDOutMin=[]  SumDOutMax=[]  SaturationOutMin=[]  SaturationOutMax=[]  IntegratorContinuousStateAttributes=''  IntegratorStateMustResolveToSignalObject=off  IntegratorRTWStateStorageClass=Auto  FilterContinuousStateAttributes=''  FilterStateMustResolveToSignalObject=off  FilterRTWStateStorageClass=Auto  DifferentiatorICPrevScaledInput=0  DifferentiatorOutMin=[]  DifferentiatorOutMax=[]  InitialConditionSetting=Output  FilterDiffOutCoefMin=[]  FilterDiffOutCoefMax=[]  SumDenOutMin=[]  SumDenOutMax=[]  SumNumOutMin=[]  SumNumOutMax=[]  ReciprocalOutMin=[]  ReciprocalOutMax=[]  DivideOutMin=[]  DivideOutMax=[]  TunerSelectOption=Transfer Function Based (PID Tuner App)
  pitchrate_setpoint : Outport
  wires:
  pitch_angle/1 -> Discrete D Controller/1
  pitch_error/1 -> Discrete PI Controller/1
  Discrete PI Controller/1 -> Add/1
  Discrete D Controller/1 -> Add/2
  Add/1 -> pitchrate_setpoint/1

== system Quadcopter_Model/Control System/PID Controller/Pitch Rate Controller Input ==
  note: 1) Add Subsystem or Model blocks as valid variant choices. 2) You cannot connect blocks at this level. At simulation, connectivity is automatically determined, based on the active variant and port name matching.
  pitchrate_error_model : Inport
  pitchrate_model : Inport  Port=2
  Feedback : Subsystem  VariantControl=logAnalysisToggle==0
  pitchrate error : Subsystem  VariantControl=logAnalysisToggle==1
  pitchrate_error : Outport
  pitchrate : Outport  Port=2

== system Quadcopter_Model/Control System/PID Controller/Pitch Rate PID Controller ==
  pitchrate_error : Inport
  pitchrate : Inport  Port=2
  Add : Sum  Inputs=+-
  Discrete D Controller : Derivative/Discrete D Controller  Kd=Kd  a=a
  Discrete PI Controller : simulink/Continuous/PID Controller  Controller=PI  TimeDomain=Discrete-time  SampleTime=Ts  IntegratorMethod=Forward Euler  FilterMethod=Forward Euler  Form=Parallel  UseFilter=on  ControllerParametersSource=internal  P=Kp  I=Ki  D=0  N=100  InitialConditionSource=internal  InitialConditionForIntegrator=0  InitialConditionForFilter=0  ExternalReset=none  LimitOutput=off  UpperSaturationLimit=inf  LowerSaturationLimit=-inf  LinearizeAsGain=off  AntiWindupMode=none  Kb=1  TrackingMode=off  Kt=1  PParamMin=[]  PParamMax=[]  IParamMin=[]  IParamMax=[]  DParamMin=[]  DParamMax=[]  NParamMin=[]  NParamMax=[]  KbParamMin=[]  KbParamMax=[]  KtParamMin=[]  KtParamMax=[]  POutMin=[]  POutMax=[]  IOutMin=[]  IOutMax=[]  DOutMin=[]  DOutMax=[]  NOutMin=[]  NOutMax=[]  KbOutMin=[]  KbOutMax=[]  KtOutMin=[]  KtOutMax=[]  IntegratorOutMin=[]  IntegratorOutMax=[]  FilterOutMin=[]  FilterOutMax=[]  SumOutMin=[]  SumOutMax=[]  SumI1OutMin=[]  SumI1OutMax=[]  SumI2OutMin=[]  SumI2OutMax=[]  SumI3OutMin=[]  SumI3OutMax=[]  SumDOutMin=[]  SumDOutMax=[]  SaturationOutMin=[]  SaturationOutMax=[]  IntegratorContinuousStateAttributes=''  IntegratorStateMustResolveToSignalObject=off  IntegratorRTWStateStorageClass=Auto  FilterContinuousStateAttributes=''  FilterStateMustResolveToSignalObject=off  FilterRTWStateStorageClass=Auto  DifferentiatorICPrevScaledInput=0  DifferentiatorOutMin=[]  DifferentiatorOutMax=[]  FilterDiffOutCoefMin=[]  FilterDiffOutCoefMax=[]  SumDenOutMin=[]  SumDenOutMax=[]  SumNumOutMin=[]  SumNumOutMax=[]  ReciprocalOutMin=[]  ReciprocalOutMax=[]  DivideOutMin=[]  DivideOutMax=[]  TunerSelectOption=Transfer Function Based (PID Tuner App)
  x_motor_command : Outport
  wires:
  pitchrate/1 -> Discrete D Controller/1
  pitchrate_error/1 -> Discrete PI Controller/1
  Discrete PI Controller/1 -> Add/1
  Discrete D Controller/1 -> Add/2
  Add/1 -> x_motor_command/1

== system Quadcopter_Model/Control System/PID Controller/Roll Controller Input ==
  note: 1) Add Subsystem or Model blocks as valid variant choices. 2) You cannot connect blocks at this level. At simulation, connectivity is automatically determined, based on the active variant and port name matching.
  roll_error_model : Inport
  roll_angle_model : Inport  Port=2
  Feedback : Subsystem  VariantControl=logAnalysisToggle==0
  roll error : Subsystem  VariantControl=logAnalysisToggle==1
  roll_error : Outport
  roll_angle : Outport  Port=2

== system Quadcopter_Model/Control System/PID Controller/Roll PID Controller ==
  roll_error : Inport
  roll_angle : Inport  Port=2
  Add : Sum  Inputs=+-
  Discrete D Controller : Derivative/Discrete D Controller  Kd=Kd  a=a
  Discrete PI Controller : simulink/Continuous/PID Controller  Controller=PI  TimeDomain=Discrete-time  SampleTime=Ts  IntegratorMethod=Forward Euler  FilterMethod=Forward Euler  Form=Parallel  UseFilter=on  ControllerParametersSource=internal  P=Kp  I=Ki  D=0  N=100  InitialConditionSource=internal  InitialConditionForIntegrator=0  InitialConditionForFilter=0  ExternalReset=none  LimitOutput=off  UpperSaturationLimit=inf  LowerSaturationLimit=-inf  LinearizeAsGain=off  AntiWindupMode=none  Kb=1  TrackingMode=off  Kt=1  PParamMin=[]  PParamMax=[]  IParamMin=[]  IParamMax=[]  DParamMin=[]  DParamMax=[]  NParamMin=[]  NParamMax=[]  KbParamMin=[]  KbParamMax=[]  KtParamMin=[]  KtParamMax=[]  POutMin=[]  POutMax=[]  IOutMin=[]  IOutMax=[]  DOutMin=[]  DOutMax=[]  NOutMin=[]  NOutMax=[]  KbOutMin=[]  KbOutMax=[]  KtOutMin=[]  KtOutMax=[]  IntegratorOutMin=[]  IntegratorOutMax=[]  FilterOutMin=[]  FilterOutMax=[]  SumOutMin=[]  SumOutMax=[]  SumI1OutMin=[]  SumI1OutMax=[]  SumI2OutMin=[]  SumI2OutMax=[]  SumI3OutMin=[]  SumI3OutMax=[]  SumDOutMin=[]  SumDOutMax=[]  SaturationOutMin=[]  SaturationOutMax=[]  IntegratorContinuousStateAttributes=''  IntegratorStateMustResolveToSignalObject=off  IntegratorRTWStateStorageClass=Auto  FilterContinuousStateAttributes=''  FilterStateMustResolveToSignalObject=off  FilterRTWStateStorageClass=Auto  DifferentiatorICPrevScaledInput=0  DifferentiatorOutMin=[]  DifferentiatorOutMax=[]  FilterDiffOutCoefMin=[]  FilterDiffOutCoefMax=[]  SumDenOutMin=[]  SumDenOutMax=[]  SumNumOutMin=[]  SumNumOutMax=[]  ReciprocalOutMin=[]  ReciprocalOutMax=[]  DivideOutMin=[]  DivideOutMax=[]  TunerSelectOption=Transfer Function Based (PID Tuner App)
  rollrate_setpoint : Outport
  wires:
  roll_angle/1 -> Discrete D Controller/1
  roll_error/1 -> Discrete PI Controller/1
  Discrete PI Controller/1 -> Add/1
  Discrete D Controller/1 -> Add/2
  Add/1 -> rollrate_setpoint/1

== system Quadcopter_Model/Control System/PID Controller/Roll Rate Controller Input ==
  note: 1) Add Subsystem or Model blocks as valid variant choices. 2) You cannot connect blocks at this level. At simulation, connectivity is automatically determined, based on the active variant and port name matching.
  rollrate_error_model : Inport
  rollrate_model : Inport  Port=2
  Feedback : Subsystem  VariantControl=logAnalysisToggle==0
  rollrate error : Subsystem  VariantControl=logAnalysisToggle==1
  rollrate_error : Outport
  rollrate : Outport  Port=2
